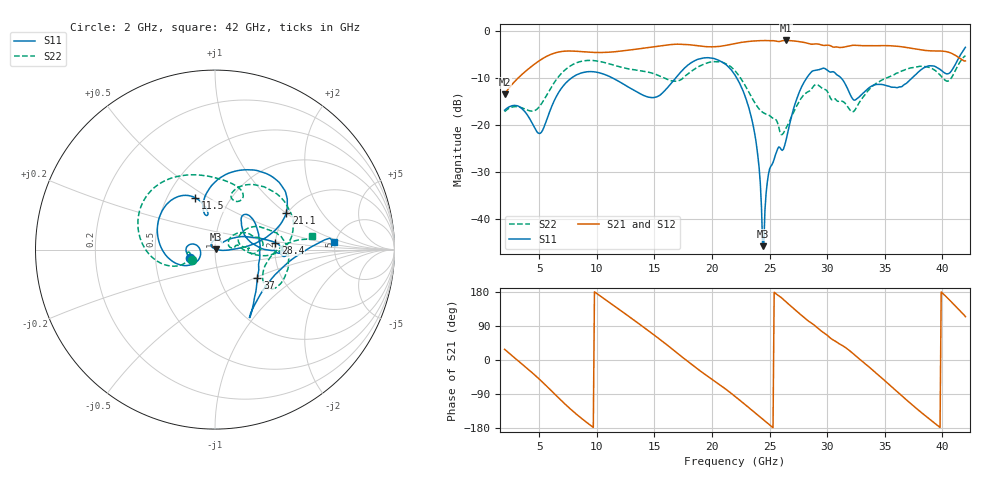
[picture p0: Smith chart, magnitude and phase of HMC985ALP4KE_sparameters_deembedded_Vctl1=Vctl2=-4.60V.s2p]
!s2p File: Measurements: S11, S21, S12, S22
# GHz S dB R 50.0
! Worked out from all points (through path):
!   401 points, 2 GHz to 42 GHz, reference 50 ohm
!   highest |S21| = -2.06 dB at 26.4 GHz (marker M1); lowest = -13.4 dB at 2 GHz (marker M2)
!   lowest |S11| = -45.7 dB at 24.4 GHz (marker M3), VSWR 1.01, Z = 50.5 + j0.143 ohm
!   |S11| at or under -10 dB: start of sweep to 7.818 GHz; 22.15 GHz to 28.23 GHz (6.083 GHz wide, 24.2 % of centre); 31.21 GHz to 37.38 GHz (6.174 GHz wide, 18 % of centre)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
!   |S22| runs from -22.0 to -5.3 dB; largest |S21 - S12| = 0.0008
!   S11 on the Smith chart (normalised r, x): 2 GHz: 0.76, -0.07; 11.5 GHz: 0.69, +0.44; 21.1 GHz: 1.97, +1.01; 28.4 GHz: 2.00, +0.18; 37 GHz: 1.51, -0.53; 42 GHz: 4.89, +0.75
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2  -16.85 -161.8  -13.44 28.2  -13.44 28.2  -17.15 -155.6
5  -21.79 -173.0  -6.38 -50.2  -6.38 -50.2  -16.14 -160.0
6.3  -14.87 -150.5  -4.76 -88.4  -4.76 -88.4  -11.02 -161.8
8.7  -8.93 150.2  -4.44 -154.7  -4.44 -154.7  -6.46 151.1
11.5  -10.19 111.0  -4.47 143.0  -4.47 143.0  -7.31 104.9
13.6  -13.14 101.3  -3.85 97.0  -3.85 97.0  -8.42 75.5
15.4  -13.79 106.1  -3.25 56.2  -3.25 56.2  -9.53 62.0
17.9  -7.30 80.1  -2.94 -3.8  -2.95 -3.8  -9.17 72.0
21.1  -6.99 27.4  -3.15 -74.7  -3.15 -74.7  -6.88 15.8
22  -9.39 16.9  -2.71 -95.9  -2.71 -95.9  -8.49 0.3
23.6  -20.38 0.4  -2.18 -135.6  -2.18 -135.6  -14.79 -4.3
24  -26.89 -5.6  -2.11 -145.6  -2.11 -145.6  -16.30 1.4
24.4  -45.67 15.8  -2.08 -155.8  -2.08 -155.7  -17.29 7.3
25.1  -28.76 125.1  -2.12 -173.5  -2.12 -173.5  -18.17 10.9
26.4  -23.52 41.6  -2.06 154.2  -2.06 154.2  -20.83 33.1
28.4  -9.40 6.6  -2.72 102.2  -2.72 102.2  -12.86 18.0
28.7  -8.58 1.7  -2.86 96.0  -2.86 96.0  -12.18 16.2
32.5  -14.59 32.5  -3.10 10.3  -3.10 10.3  -16.47 28.0
35.4  -11.79 18.8  -3.17 -65.2  -3.17 -65.2  -9.77 19.2
37  -10.88 -34.1  -3.59 -108.3  -3.60 -108.3  -8.06 4.7
39.8  -8.19 -57.2  -4.29 -178.0  -4.30 -178.0  -9.38 -35.6
42  -3.52 3.7  -6.40 114.3  -6.41 114.3  -5.26 8.2
